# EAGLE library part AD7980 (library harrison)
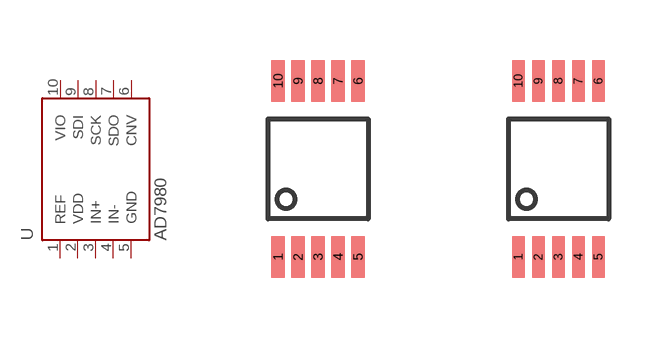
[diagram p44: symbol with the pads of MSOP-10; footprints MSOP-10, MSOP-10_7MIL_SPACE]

Designator prefix U

## AD7980-MSOP  [MSOP-10]
1  REF  in
2  VDD  pwr
3  IN+  in
4  IN-  in
5  GND  pwr
6  CNV  in
7  SDO  out
8  SCK  in
9  SDI  in
10  VIO  pwr

## AD7980-MSOP-7MIL  [MSOP-10_7MIL_SPACE]
Pads as for MSOP-10

## Footprint MSOP-10 (pad centres in mm)
smd 0.34 x 1.04: 1 -1,-2.2; 2 -0.5,-2.2; 3 0,-2.2; 4 0.5,-2.2; 5 1,-2.2; 6 1,2.2; 7 0.5,2.2; 8 0,2.2; 9 -0.5,2.2; 10 -1,2.2

## Footprint MSOP-10_7MIL_SPACE (pad centres in mm)
smd 0.32 x 1.04: 1 -1,-2.2; 2 -0.5,-2.2; 3 0,-2.2; 4 0.5,-2.2; 5 1,-2.2; 6 1,2.2; 7 0.5,2.2; 8 0,2.2; 9 -0.5,2.2; 10 -1,2.2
